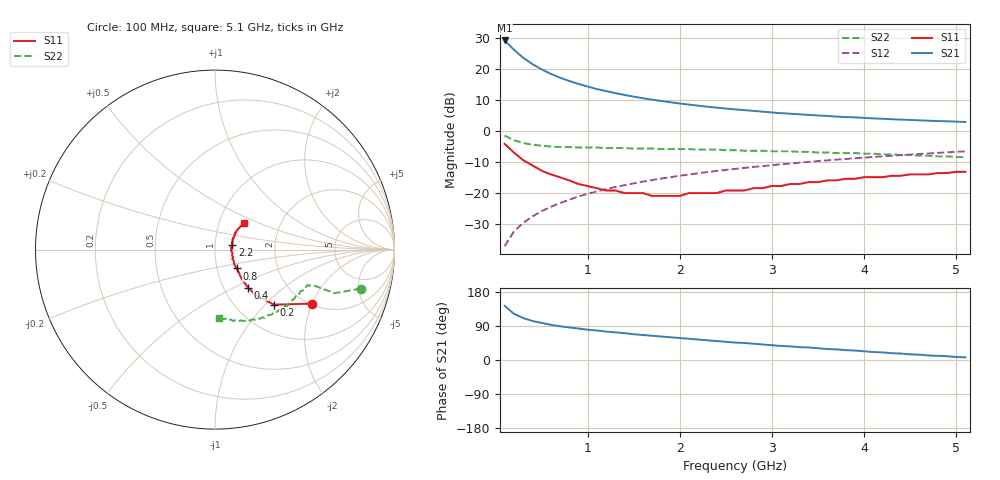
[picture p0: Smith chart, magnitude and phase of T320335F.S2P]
!AT-32033
!S PARAMETERS at Vce=5 V  Ic=15mA.  LAST UPDATED 01-05-95
# ghz s ma r 50
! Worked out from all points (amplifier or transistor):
!   51 points, 100 MHz to 5.1 GHz, reference 50 ohm
!   highest |S21| = 29.1 dB at 100 MHz (marker M1)
!   |S21| within 3 dB of that: start of sweep to 201.7 MHz
!   unconditionally stable (mu >= 1): 865.1 MHz to 2.098 GHz; 2.101 GHz to 2.252 GHz
!   at 900 MHz: K = 1.00, MAG = 17.9 dB, |S12| = -21.1 dB
!   at 2.6 GHz: K = 0.99, MSG = 9.6 dB, |S12| = -12.2 dB
!   at 5.1 GHz: K = 0.94, MSG = 4.7 dB, |S12| = -6.6 dB
!   S11 on the Smith chart (normalised r, x): 100 MHz: 2.05, -2.00; 200 MHz: 1.47, -1.13; 400 MHz: 1.30, -0.59; 800 MHz: 1.24, -0.27; 2.2 GHz: 1.21, +0.06; 5.1 GHz: 1.31, +0.41
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0.1  0.62 -29.0  28.5 143.0  0.014 77.0  0.84 -15.0
0.2  0.45 -43.0  20.28 122.0  0.024 75.0  0.71 -20.0
0.3  0.34 -48.0  15.11 111.0  0.033 75.0  0.64 -20.0
0.4  0.28 -49.0  11.91 103.0  0.042 75.0  0.6 -20.0
0.5  0.23 -48.0  9.79 98.0  0.051 75.0  0.58 -20.0
0.6  0.2 -46.0  8.3 93.0  0.06 75.0  0.56 -21.0
0.7  0.18 -43.0  7.2 89.0  0.069 75.0  0.55 -21.0
0.8  0.16 -41.0  6.36 86.0  0.078 75.0  0.55 -22.0
0.9  0.14 -38.0  5.71 83.0  0.088 74.0  0.54 -23.0
1  0.13 -36.0  5.18 80.0  0.097 73.0  0.54 -24.0
1.1  0.12 -30.0  4.72 78.0  0.106 72.0  0.54 -25.0
1.2  0.11 -29.0  4.37 75.0  0.116 72.0  0.53 -26.0
1.3  0.11 -23.0  4.06 73.0  0.125 71.0  0.53 -27.0
1.5  0.1 -14.0  3.56 68.0  0.143 69.0  0.52 -30.0
1.8  0.09 -1.0  3.03 62.0  0.171 66.0  0.51 -34.0
2  0.09 8.0  2.76 58.0  0.19 64.0  0.51 -36.0
2.2  0.1 15.0  2.55 54.0  0.208 62.0  0.5 -39.0
2.6  0.11 27.0  2.22 46.0  0.245 58.0  0.49 -45.0
3.1  0.13 35.0  1.93 37.0  0.29 52.0  0.47 -52.0
3.5  0.15 40.0  1.77 31.0  0.327 48.0  0.45 -58.0
4.3  0.19 42.0  1.54 18.0  0.399 40.0  0.42 -72.0
5.1  0.22 43.0  1.39 7.0  0.469 31.0  0.38 -87.0
